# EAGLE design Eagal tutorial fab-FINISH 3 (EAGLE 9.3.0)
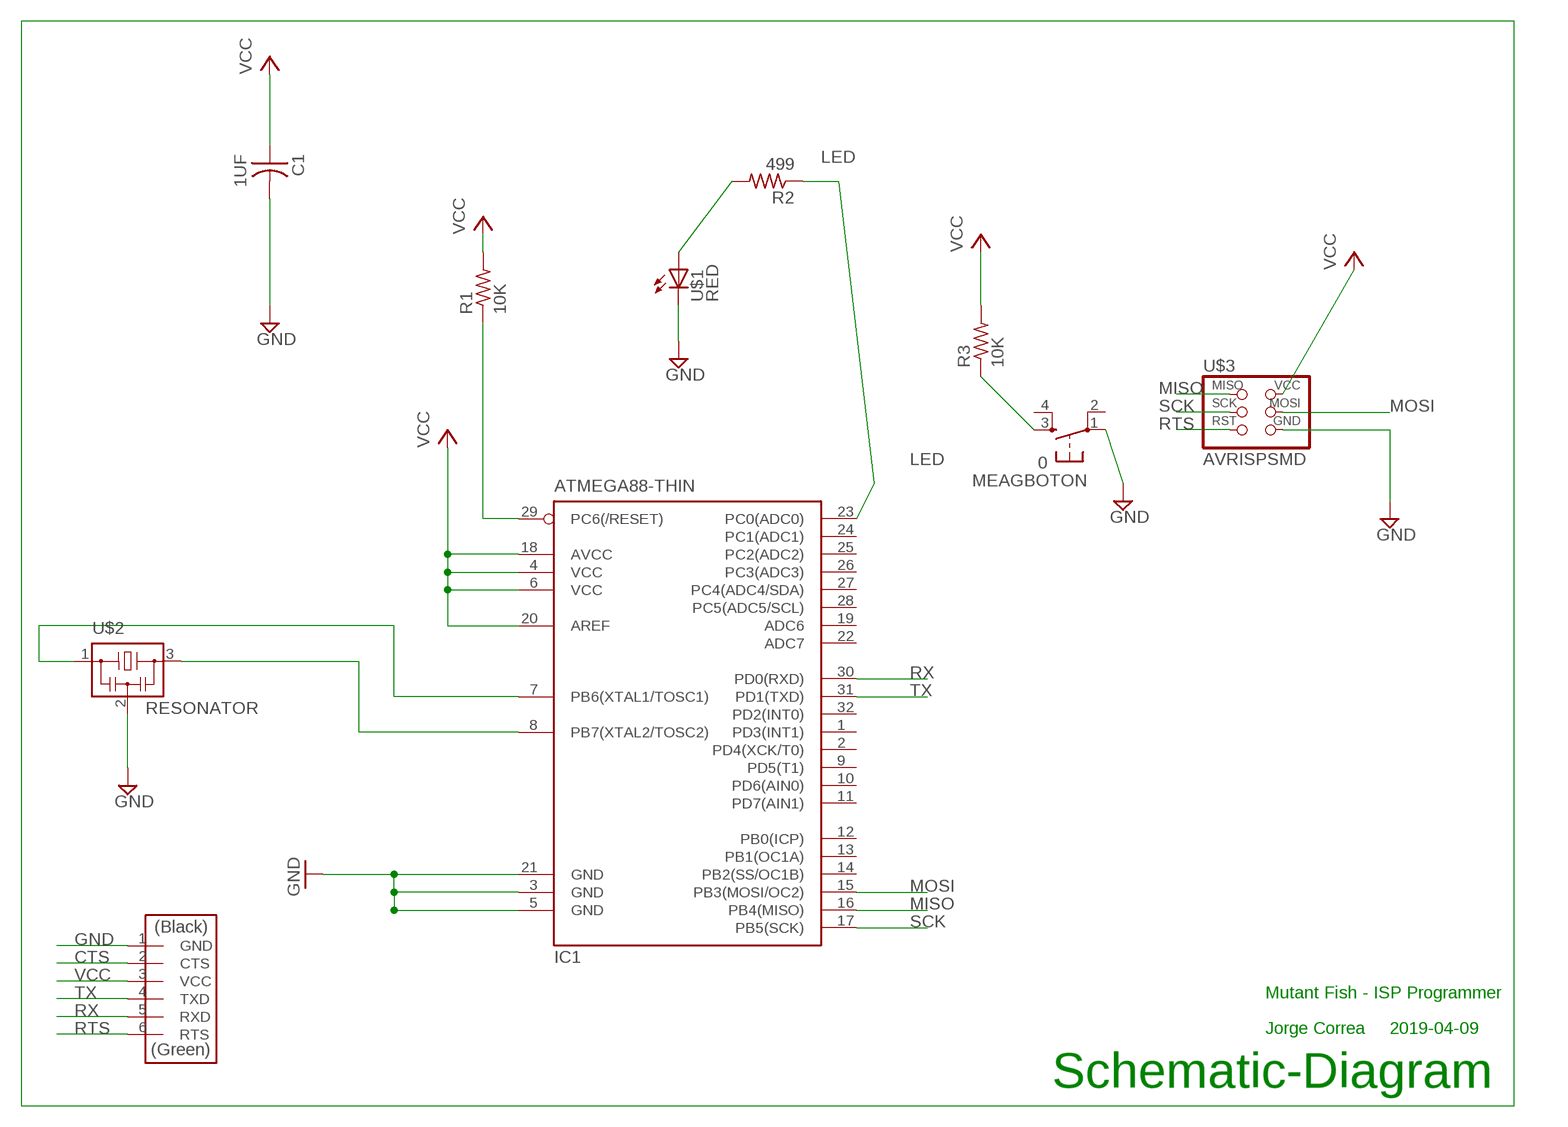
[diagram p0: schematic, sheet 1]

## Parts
C1  1UF  CAP-US1206FAB  [C1206FAB]
IC1  ATMEGA88-THIN  [TQFP32-08THIN]
MEAGBOTON  0  6MM_SWITCH6MM_SWITCH  [6MM_SWITCH]
R1  10K  RES-US1206FAB  [R1206FAB]
R2  499  RES-US1206FAB  [R1206FAB]
R3  10K  RES-US1206FAB  [R1206FAB]
U$1  RED  LEDFAB1206  [LED1206FAB]
U$2  RESONATOR  [EFOBM]
U$3  AVRISPSMD  [2X03SMD]
U$4  FTDI-SMD-HEADER  [1X06SMD]

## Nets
CTS: U$4.2(CTS)
GND: C1.2 IC1.3(GND) IC1.5(GND) IC1.21(GND) MEAGBOTON.1(P) U$1.2(C) U$2.2 U$3.6(GND) U$4.1(GND)
LED: IC1.23(PC0(ADC0)) R2.1
MISO: IC1.16(PB4(MISO)) U$3.1(MISO)
MOSI: IC1.15(PB3(MOSI/OC2)) U$3.4(MOSI)
N$1: IC1.8(PB7(XTAL2/TOSC2)) U$2.3
N$2: IC1.7(PB6(XTAL1/TOSC1)) U$2.1
N$3: IC1.29(PC6(/RESET)) R1.1
N$4: R2.2 U$1.1(A)
N$5: MEAGBOTON.3(S) R3.1
RTS: U$3.5(RST) U$4.6(RTS)
RX: IC1.30(PD0(RXD)) U$4.5(RXD)
SCK: IC1.17(PB5(SCK)) U$3.3(SCK)
TX: IC1.31(PD1(TXD)) U$4.4(TXD)
VCC: C1.1 IC1.4(VCC) IC1.6(VCC) IC1.18(AVCC) IC1.20(AREF) R1.2 R3.2 U$3.2(VCC) U$4.3(VCC)
Unconnected: IC1.1(PD3(INT1)) IC1.2(PD4(XCK/T0)) IC1.9(PD5(T1)) IC1.10(PD6(AIN0)) IC1.11(PD7(AIN1)) IC1.12(PB0(ICP)) IC1.13(PB1(OC1A)) IC1.14(PB2(SS/OC1B)) IC1.19(ADC6) IC1.22(ADC7) IC1.24(PC1(ADC1)) IC1.25(PC2(ADC2)) IC1.26(PC3(ADC3)) IC1.27(PC4(ADC4/SDA)) IC1.28(PC5(ADC5/SCL)) IC1.32(PD2(INT0)) MEAGBOTON.2(P1) MEAGBOTON.4(S1)

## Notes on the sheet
- Mutant Fish - ISP Programmer
- Jorge Correa | 2019-04-09
- Schematic-Diagram

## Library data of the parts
C1 = fab:CAP-US
IC1 = fab:ATMEGA88-THIN
MEAGBOTON = fab:6MM_SWITCH: OMRON SWITCH
R1-R3 = fab:RES-US: Resistor (US Symbol)
U$1 = fab:LED: LED
U$2 = fab:RESONATOR
U$3 = fab:AVRISP
U$4 = fab:FTDI-SMD-HEADER

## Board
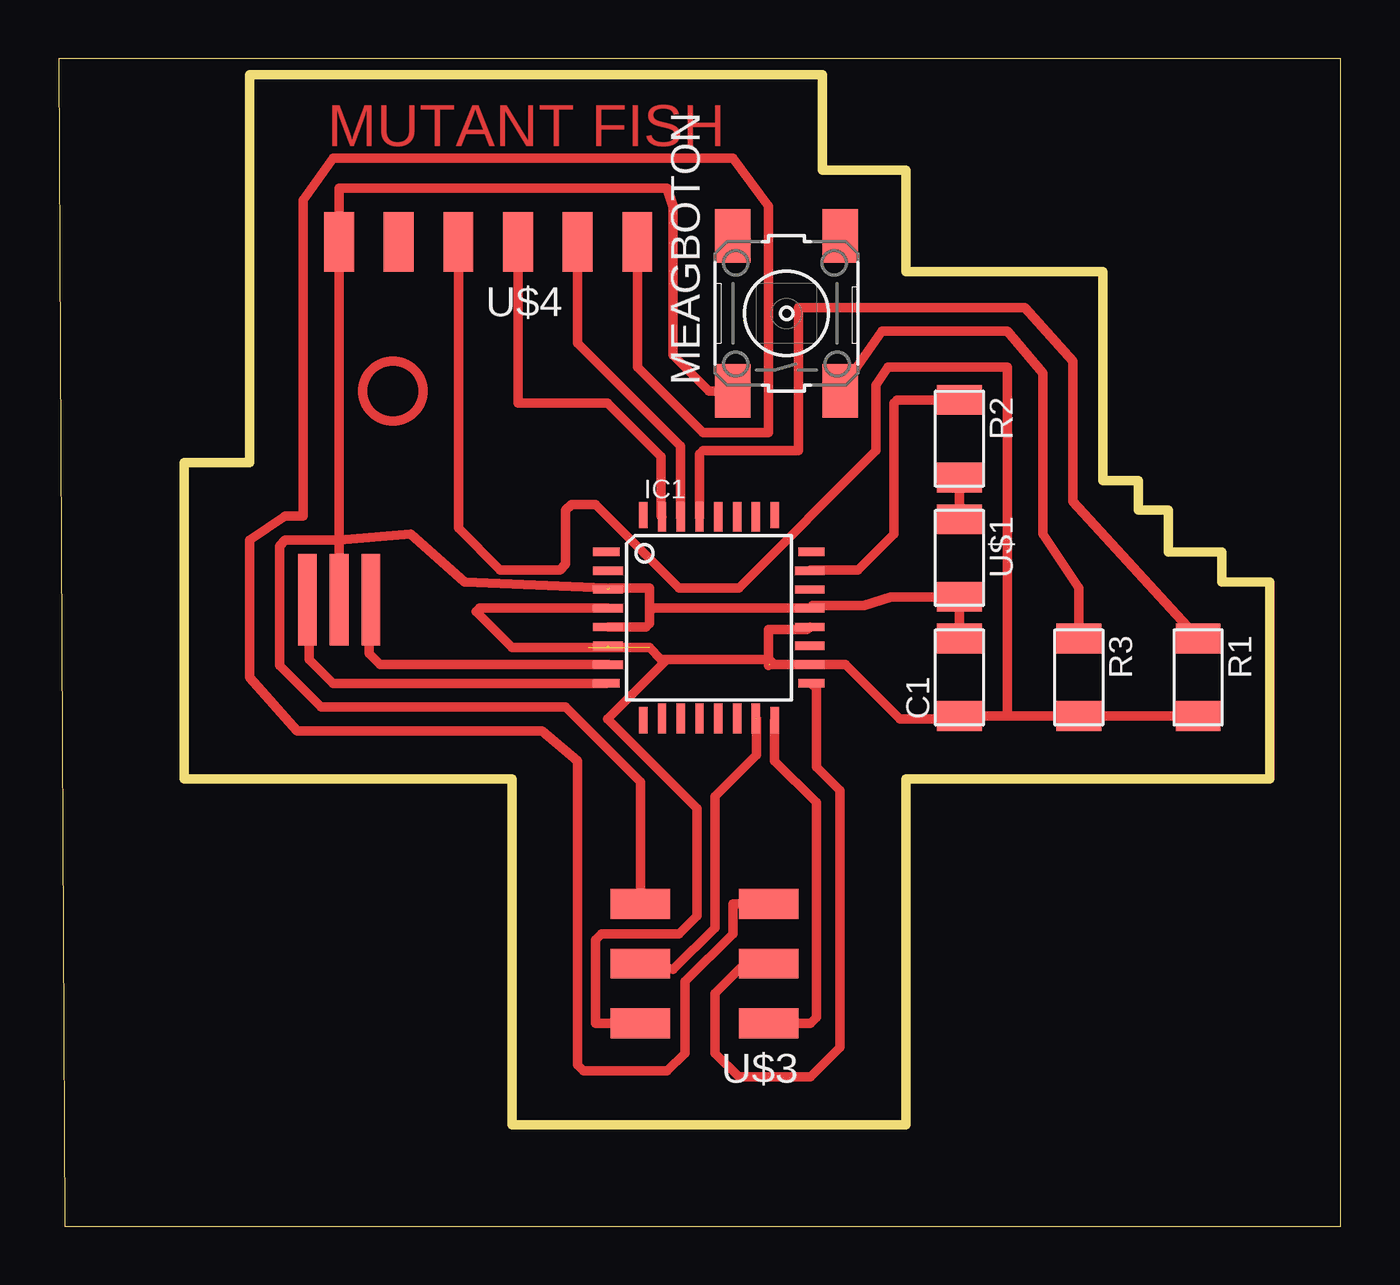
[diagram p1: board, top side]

Size 54.59 x 49.71 mm. Coordinates in mm from the lower left corner, seen from the top.
Outline: 0.25,0 54.59,0 54.59,49.71 0,49.71 0.25,0
Copper layers (1*16): Top 0.035mm / dielectric 1.5mm / Bottom 0.035mm
Design rules "default": minimum track width 10mil, minimum drill 24mil, track to track 8mil, track to pad 8mil, pad to pad 8mil, via to via 8mil, smd to smd 8mil, copper to edge 40mil, drill to drill 8mil, minimum pad ring 10mil, minimum via ring 8mil, stop-mask expansion 4mil, vias tented up to drill 0mil, thermal gap 10mil
Milling: 24 lines

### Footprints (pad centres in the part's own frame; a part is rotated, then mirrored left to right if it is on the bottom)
C1206FAB = smd 1.27 x 1.905: 1 -1.651,0; 2 1.651,0
TQFP32-08THIN = smd 1.118 x 0.356: 1 -4.369,2.8; 8 -4.369,-2.8; 17 4.369,-2.8; 24 4.369,2.8 | smd 1.27 x 0.356: 2 -4.293,2; 3 -4.293,1.2; 4 -4.293,0.4; 5 -4.293,-0.4; 6 -4.293,-1.2; 7 -4.293,-2; 18 4.293,-2; 19 4.293,-1.2; 20 4.293,-0.4; 21 4.293,0.4; 22 4.293,1.2; 23 4.293,2 | smd 0.356 x 1.118: 9 -2.8,-4.369; 16 2.8,-4.369; 25 2.8,4.369; 32 -2.8,4.369 | smd 0.356 x 1.27: 10 -2,-4.293; 14 1.2,-4.293; 15 2,-4.293; 26 2,4.293; 27 1.2,4.293; 31 -2,4.293 | smd 0.35 x 1.27: 11 -1.2,-4.293; 12 -0.4,-4.293; 13 0.4,-4.293; 28 0.4,4.293; 29 -0.4,4.293; 30 -1.2,4.293
6MM_SWITCH = smd 2.286 x 1.524: 1 -3.302,2.286; 2 3.302,2.286; 3 -3.302,-2.286; 4 3.302,-2.286
R1206FAB = smd 1.27 x 1.905: 1 -1.651,0; 2 1.651,0
LED1206FAB = smd 1.27 x 1.905: 1 -1.651,0; 2 1.651,0
EFOBM = smd 0.8 x 3.9: 1 -1.35,0; 2 0,0; 3 1.35,0
2X03SMD = smd 2.54 x 1.27: 1 -2.54,2.54; 2 2.92,2.54; 3 -2.54,0; 4 2.92,0; 5 -2.54,-2.54; 6 2.92,-2.54
1X06SMD = smd 2.54 x 1.27: 1 0,6.35; 2 0,3.81; 3 0,1.27; 4 0,-1.27; 5 0,-3.81; 6 0,-6.35

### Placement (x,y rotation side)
C1  38.35,23.37 90 top
IC1  27.69,25.91 0 top
MEAGBOTON  30.99,38.86 90 top
R1  48.51,23.37 270 top
R2  38.35,33.53 270 top
R3  43.43,23.37 270 top
U$1  38.35,28.45 270 top
U$2  11.94,26.67 180 top
U$3  27.69,11.18 180 top
U$4  18.29,41.91 90 top

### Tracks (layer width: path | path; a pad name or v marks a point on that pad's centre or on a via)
GND  (2 unrouted)
  Top 0.406: 11.94,29.21 U$4.1 11.94,44.2 25.91,44.2 26.16,43.43 26.16,37.08 27.69,35.56 MEAGBOTON.1 | U$2.2 11.94,29.21 | 11.94,29.21 14.99,29.46 17.27,27.43 23.32,27.18 | U$3.6 24.77,18.92 21.59,22.1 11.18,22.1 9.4,23.88 9.4,28.96 9.65,29.21 11.94,29.21 | C1.2 U$1.2 35.43,26.8 34.29,26.42 32.09,26.42 IC1.21 25.29,26.31 25.15,26.16 | IC1.5 25,25.51 25.15,25.65 25.15,26.16 | 25.15,26.16 25.15,27.18 23.46,27.18
LED
  Top 0.406: R2.1 35.69,35.18 35.56,35.05 35.56,29.46 34.04,27.94 32.01,27.94 IC1.23
MISO
  Top 0.406: U$3.1 32,8.64 32.26,8.89 32.26,18.03 30.48,19.81 30.48,21.53 IC1.16
MOSI  (1 unrouted)
  Top 0.406: U$3.4 26.16,10.92 27.94,12.7 27.94,18.29 29.72,20.07 29.72,21.58
N$1
  Top 0.406: IC1.8 11.69,23.11 10.67,24.13 10.67,26.59 U$2.3
N$2
  Top 0.406: IC1.7 13.68,23.91 13.21,24.38 13.21,26.59 U$2.1
N$3
  Top 0.406: IC1.29 27.29,32.87 27.43,33.02 31.5,33.02 31.5,39.12 41.15,39.12 43.18,36.83 43.18,30.86 R1.1
N$4
  Top 0.406: U$1.1 R2.2
N$5
  Top 0.406: R3.1 43.43,27.18 41.91,29.46 41.91,36.32 40.39,38.1 35.05,38.1 MEAGBOTON.3
RTS
  Top 0.406: U$4.6 24.64,36.58 27.43,33.78 30.23,33.78 30.23,43.43 28.7,45.47 11.68,45.47 10.41,43.69 10.41,30.23 9.65,30.23 8.13,29.21 8.13,23.37 10.16,21.08 20.57,21.08 22.1,19.81 22.1,6.86 22.35,6.6 25.91,6.6 26.67,7.37 26.67,10.41 28.7,12.45 28.7,13.72 U$3.5
RX
  Top 0.406: IC1.30 26.49,33.2 22.1,37.59 U$4.5
SCK
  Top 0.406: U$3.3 29.21,11.18 27.94,9.91 27.94,7.37 28.96,6.35 32,6.35 33.27,7.62 33.27,18.54 32.26,19.56 32.26,22.9 IC1.17
TX
  Top 0.406: U$4.4 19.56,35.05 23.37,35.05 25.65,32.77 25.65,30.23 IC1.31
VCC  (6 unrouted)
  Top 0.406: 40.39,21.72 C1.1 38.23,21.59 35.81,21.59 33.5,23.91 IC1.18 30.48,23.91 | 40.39,21.72 R3.2 R1.2 | 30.48,23.91 30.26,23.91 | 30.23,23.88 30.23,25.4 31.87,25.4 IC1.20 | U$3.2 22.86,8.64 22.86,12.19 23.11,12.45 26.42,12.45 27.18,13.21 27.18,17.78 23.37,21.59 25.91,24.13 | 25.91,24.13 30.26,24.13 30.48,23.91 | 25.91,24.13 25.65,24.13 25.15,24.64 19.3,24.64 17.78,26.16 17.93,26.31 IC1.4 | U$4.3 17.02,29.72 18.8,27.94 21.34,27.94 21.59,28.19 21.59,30.48 21.84,30.73 22.86,30.73 26.42,27.18 28.96,27.18 34.8,33.02 34.8,35.81 35.31,36.58 40.39,36.58 40.39,21.72
(copper drawn outside any net)
  shapes: Top circle x1

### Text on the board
Top: MUTANT FISH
